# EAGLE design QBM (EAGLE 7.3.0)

## Sheet 1 of 3: dual 1 -> 2 mult
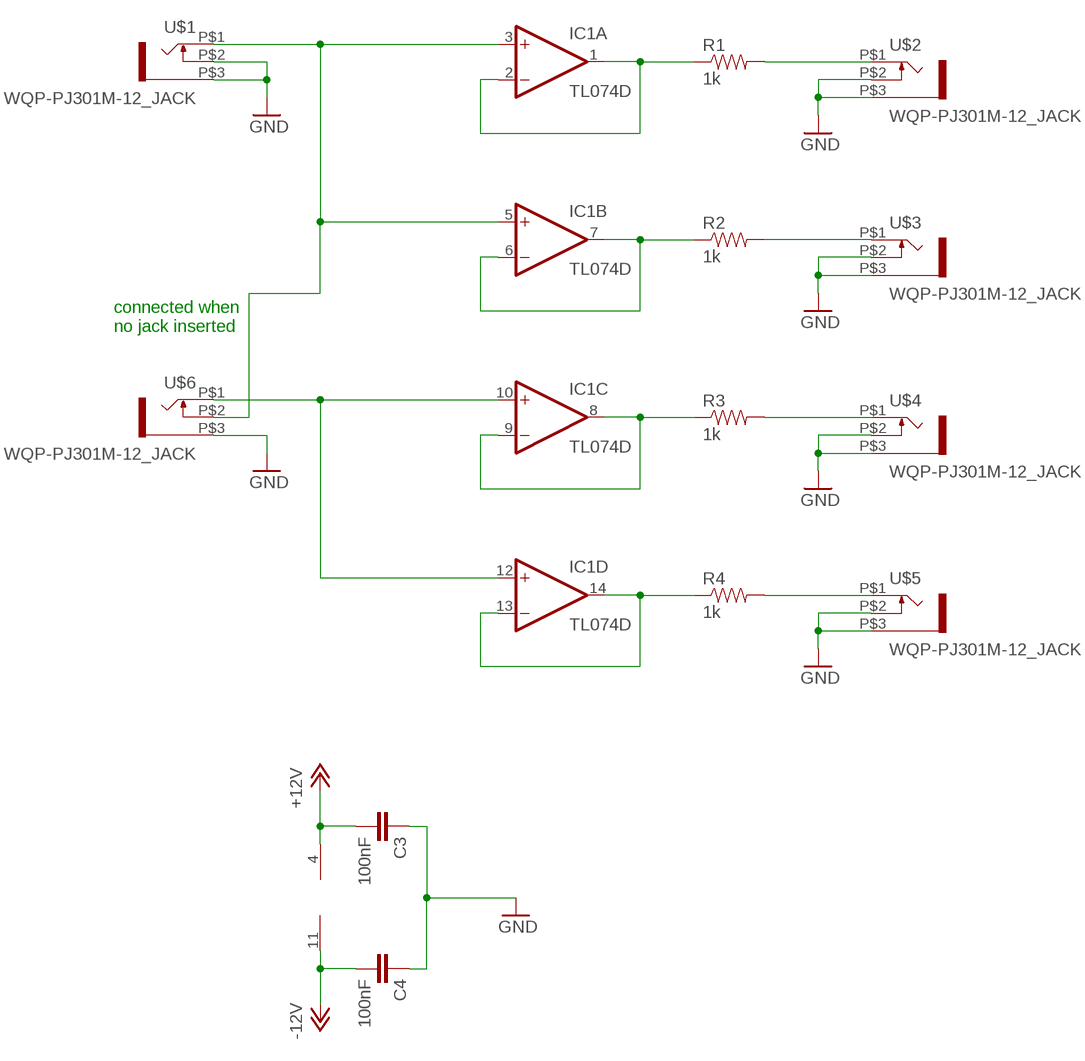
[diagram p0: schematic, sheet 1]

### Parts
C3  100nF  CAP1206  [1206]
C4  100nF  CAP1206  [1206]
IC1  TL074D  [SO14]
R1  1k  RESISTOR1206  [1206]
R2  1k  RESISTOR1206  [1206]
R3  1k  RESISTOR1206  [1206]
R4  1k  RESISTOR1206  [1206]
U$1  WQP-PJ301M-12_JACK  [WQP-PJ301M-12_JACK]
U$2  WQP-PJ301M-12_JACK  [WQP-PJ301M-12_JACK]
U$3  WQP-PJ301M-12_JACK  [WQP-PJ301M-12_JACK]
U$4  WQP-PJ301M-12_JACK  [WQP-PJ301M-12_JACK]
U$5  WQP-PJ301M-12_JACK  [WQP-PJ301M-12_JACK]
U$6  WQP-PJ301M-12_JACK  [WQP-PJ301M-12_JACK]

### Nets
+12V: C3.2 IC1.4(P:V+) ; also sheet 2,3
-12V: C4.2 IC1.11(P:V-) ; also sheet 2,3
GND: C3.1 C4.1 U$1.P$2 U$1.P$3 U$2.P$2 U$2.P$3 U$3.P$2 U$3.P$3 U$4.P$2 U$4.P$3 U$5.P$2 U$5.P$3 U$6.P$3 ; also sheet 2,3
N$3: IC1.3(A:+IN) IC1.5(B:+IN) U$1.P$1 U$6.P$2
N$4: IC1.1(A:OUT) IC1.2(A:-IN) R1.1
N$5: IC1.6(B:-IN) IC1.7(B:OUT) R2.1
N$6: IC1.8(C:OUT) IC1.9(C:-IN) R3.1
N$7: IC1.13(D:-IN) IC1.14(D:OUT) R4.1
N$8: R1.2 U$2.P$1
N$9: R2.2 U$3.P$1
N$10: R3.2 U$4.P$1
N$11: R4.2 U$5.P$1
N$12: IC1.10(C:+IN) IC1.12(D:+IN) U$6.P$1

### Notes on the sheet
- connected when 
  no jack inserted

## Sheet 2 of 3: dual 1 -> 2 mult
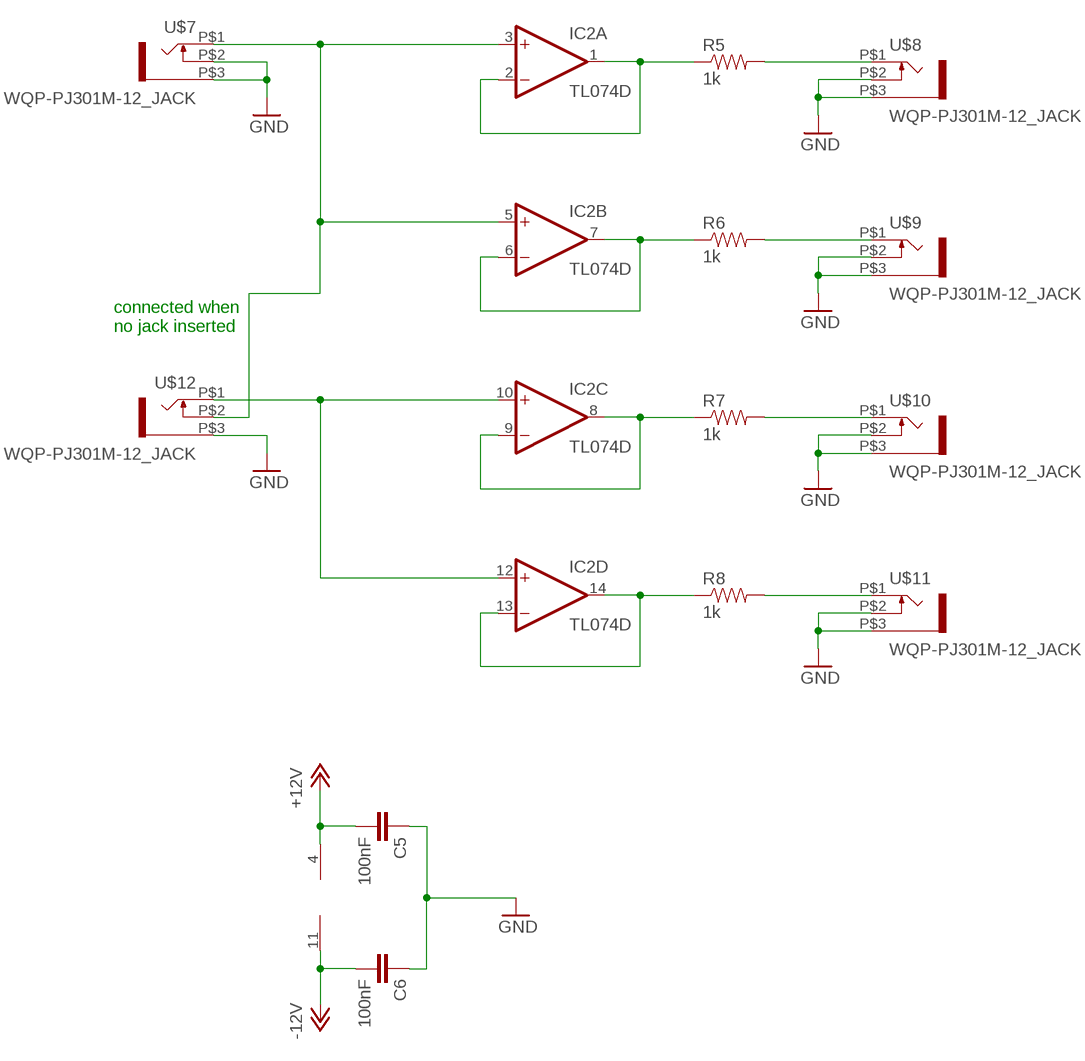
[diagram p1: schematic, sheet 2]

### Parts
C5  100nF  CAP1206  [1206]
C6  100nF  CAP1206  [1206]
IC2  TL074D  [SO14]
R5  1k  RESISTOR1206  [1206]
R6  1k  RESISTOR1206  [1206]
R7  1k  RESISTOR1206  [1206]
R8  1k  RESISTOR1206  [1206]
U$7  WQP-PJ301M-12_JACK  [WQP-PJ301M-12_JACK]
U$8  WQP-PJ301M-12_JACK  [WQP-PJ301M-12_JACK]
U$9  WQP-PJ301M-12_JACK  [WQP-PJ301M-12_JACK]
U$10  WQP-PJ301M-12_JACK  [WQP-PJ301M-12_JACK]
U$11  WQP-PJ301M-12_JACK  [WQP-PJ301M-12_JACK]
U$12  WQP-PJ301M-12_JACK  [WQP-PJ301M-12_JACK]

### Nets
+12V: C5.2 IC2.4(P:V+) ; also sheet 1,3
-12V: C6.2 IC2.11(P:V-) ; also sheet 1,3
GND: C5.1 C6.1 U$7.P$2 U$7.P$3 U$8.P$2 U$8.P$3 U$9.P$2 U$9.P$3 U$10.P$2 U$10.P$3 U$11.P$2 U$11.P$3 U$12.P$3 ; also sheet 1,3
N$13: IC2.3(A:+IN) IC2.5(B:+IN) U$7.P$1 U$12.P$2
N$14: IC2.1(A:OUT) IC2.2(A:-IN) R5.1
N$15: IC2.6(B:-IN) IC2.7(B:OUT) R6.1
N$16: IC2.8(C:OUT) IC2.9(C:-IN) R7.1
N$17: IC2.13(D:-IN) IC2.14(D:OUT) R8.1
N$18: R5.2 U$8.P$1
N$19: R6.2 U$9.P$1
N$20: R7.2 U$10.P$1
N$21: R8.2 U$11.P$1
N$22: IC2.10(C:+IN) IC2.12(D:+IN) U$12.P$1

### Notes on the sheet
- connected when 
  no jack inserted

## Sheet 3 of 3: power
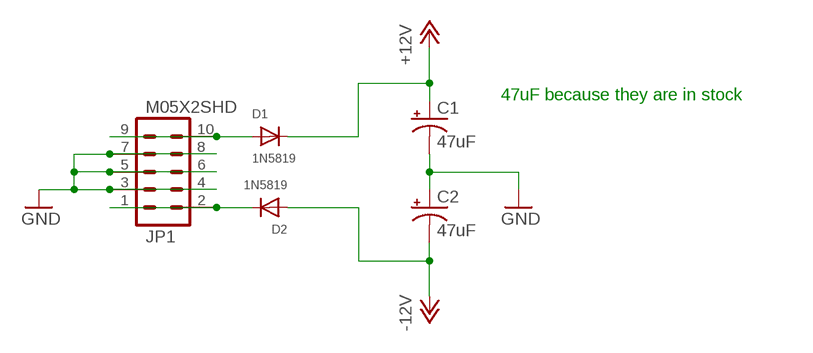
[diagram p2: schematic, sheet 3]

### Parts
C1  47uF  47UF-50V-20%(ELECT)  [PANASONIC_D]
C2  47uF  47UF-50V-20%(ELECT)  [PANASONIC_D]
D1  1N5819  DIODESOD-123  [SOD-123]
D2  1N5819  DIODESOD-123  [SOD-123]
JP1  M05X2SHD  [2X5-SHROUDED]

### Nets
+12V: C1.+ D1.C ; also sheet 1,2
-12V: C2.- D2.A ; also sheet 1,2
GND: C1.- C2.+ JP1.3 JP1.4 JP1.5 JP1.6 JP1.7 JP1.8 ; also sheet 1,2
N$1: D1.A JP1.9 JP1.10
N$2: D2.C JP1.1 JP1.2

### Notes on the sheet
- 47uF because they are in stock

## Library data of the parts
C1 C2 = SparkFun-Capacitors:47UF-50V-20%(ELECT): CAP-10547; PROD_ID: CAP-10547
C3-C6 = SparkFun-Capacitors:CAP: Capacitor
D1 D2 = adafruit:DIODE: Diode
IC1 IC2 = linear:TL074: OP AMP
JP1 = SparkFun:M05X2: Header 5x2 Standard 10-pin dual row 0.1" header. Commonly used with AVR-ISP. Use with Spark Fun Electronics SKU: PRT-00778
R1-R8 = SparkFun:RESISTOR: Resistor
U$1-U$12 = thonkiconn:WQP-PJ301M-12_JACK

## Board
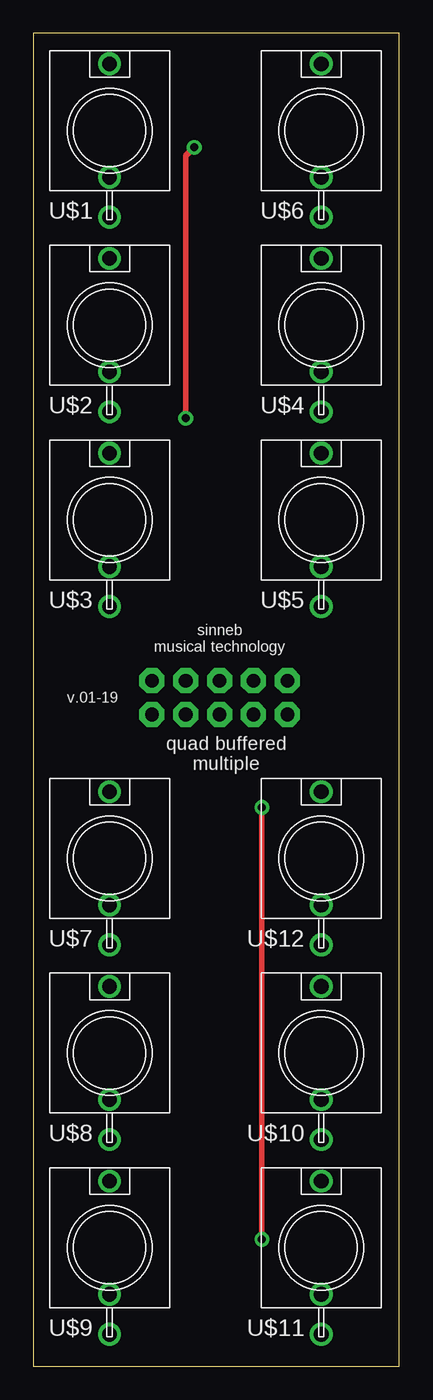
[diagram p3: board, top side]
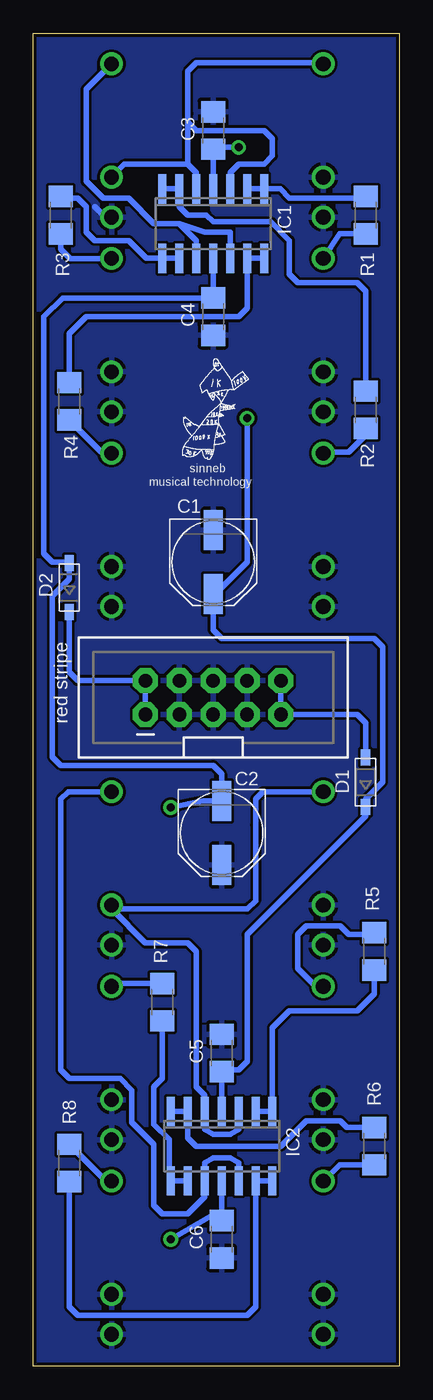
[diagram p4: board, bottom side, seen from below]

Size 27.46 x 100 mm. Coordinates in mm from the lower left corner, seen from the top.
Outline: 0,0 27.46,0 27.46,100 0,100 0,0
Copper layers (1*16): Top 0.035mm / dielectric 1.5mm / Bottom 0.035mm
Design rules "SparkFun": minimum track width 8mil, minimum drill 20mil, track to track 8mil, track to pad 8mil, pad to pad 8mil, via to via 8mil, smd to smd 8mil, copper to edge 10mil, drill to drill 8mil, minimum pad ring 12mil, minimum via ring 10mil, stop-mask expansion 4mil, vias tented up to drill 25mil, thermal gap 10mil

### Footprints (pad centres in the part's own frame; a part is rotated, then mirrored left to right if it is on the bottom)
PANASONIC_D = smd 3 x 1.4: + 2.4,0; - -2.4,0
1206 = smd 1.6 x 1.8: 1 -1.4,0; 2 1.4,0
SOD-123 = smd 1.2 x 0.7: A 1.85,0; C -1.85,0
SO14 = smd 0.6 x 2.2: 1 -3.81,-2.6; 2 -2.54,-2.6; 3 -1.27,-2.6; 4 0,-2.6; 5 1.27,-2.6; 6 2.54,-2.6; 7 3.81,-2.6; 8 3.81,2.6; 9 2.54,2.6; 10 1.27,2.6; 11 0,2.6; 12 -1.27,2.6; 13 -2.54,2.6; 14 -3.81,2.6
2X5-SHROUDED = drill 1.016 pad 1.88 octagon: 1 -1.27,5.08; 2 1.27,5.08; 3 -1.27,2.54; 4 1.27,2.54; 5 -1.27,0; 6 1.27,0; 7 -1.27,-2.54; 8 1.27,-2.54; 9 -1.27,-5.08; 10 1.27,-5.08
WQP-PJ301M-12_JACK = drill 1.1: P$1 0,5; P$2 0,-3.5; P$3 0,-6.5

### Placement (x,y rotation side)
C1  13.97,60.33 270 bottom
C2  13.34,40.01 270 bottom
C3  13.97,92.71 270 bottom
C4  13.97,78.74 90 bottom
C5  13.34,23.5 270 bottom
C6  13.34,9.53 90 bottom
D1  2.54,43.81 90 bottom
D2  24.77,58.42 90 bottom
IC1  13.97,85.72 180 bottom
IC2  13.34,16.51 180 bottom
JP1  13.97,50.16 90 bottom
R1  2.54,86.36 270 bottom
R2  2.54,71.75 270 bottom
R3  25.4,86.36 270 bottom
R4  24.77,72.39 270 bottom
R5  1.9,31.11 90 bottom
R6  1.9,16.51 270 bottom
R7  17.78,27.3 90 bottom
R8  24.77,15.24 90 bottom
U$1  5.71,92.71 0 top
U$2  5.71,78.11 0 top
U$3  5.71,63.5 0 top
U$4  21.59,78.11 0 top
U$5  21.59,63.5 0 top
U$6  21.59,92.71 0 top
U$7  5.71,38.1 0 top
U$8  5.71,23.5 0 top
U$9  5.71,8.89 0 top
U$10  21.59,23.5 0 top
U$11  21.59,8.89 0 top
U$12  21.59,38.1 0 top

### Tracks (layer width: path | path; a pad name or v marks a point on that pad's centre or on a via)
+12V  (via drill 0.6)
  Top 0.406: v11.43,71.12 11.43,90.81 v12.07,91.44
  Bottom 0.406: IC1.4 C3.2 13.84,91.44 v12.07,91.44 | IC2.4 C5.2 13.21,22.23 12.07,22.23 11.43,22.86 11.43,32.38 2.54,41.27 D1.C 2.54,42.55 1.27,43.81 1.27,53.98 1.9,54.61 13.34,54.61 13.97,55.24 C1.+ 13.83,57.92 11.43,60.33 v11.43,71.12
-12V  (via drill 0.6)
  Top 0.406: v17.14,41.91 v17.14,9.53
  Bottom 0.406: IC1.11 C4.2 25.27,80.14 26.67,78.74 26.67,60.96 26.04,60.33 24.82,60.33 D2.A 24.77,59.05 26.04,57.78 26.04,45.72 25.4,45.09 13.97,45.09 13.34,44.45 C2.- 14.75,42.41 v17.14,41.91 | IC2.11 C6.2 13.84,11.43 v17.14,9.53
GND
  Bottom 0.406: U$6.P$3 22.07,86.21 22.86,87
  pour Bottom: 0,0 0,99.69 27.3,99.69 27.3,0
N$1
  Bottom 0.406: JP1.10 JP1.9 3.18,48.9 2.54,48.26 D1.A
N$2
  Bottom 0.406: JP1.1 JP1.2 24.13,51.44 24.77,52.07 D2.C
N$3
  Bottom 0.406: IC1.5 15.24,89.53 | 15.24,89.53 15.88,90.17 | 15.88,90.17 20.63,90.17 U$6.P$2 | 15.88,93.98 15.88,93.34 15.24,92.71 12.7,92.71 10.16,92.71 9.53,92.08 9.53,90.81 10.16,90.17 12.07,90.17 12.7,89.53 IC1.3 | 15.88,93.98 15.88,97.16 15.24,97.79 6.43,97.79 U$1.P$1 | 15.24,89.53 15.88,90.17 | 15.88,90.17 15.88,93.98
N$4
  Bottom 0.406: IC1.2 IC1.1 8.95,88.33 8.26,87.63 2.67,87.63 R1.1
N$5
  Bottom 0.406: IC1.7 IC1.6 16.51,87 15.88,86.36 14.48,86.36 13.97,85.85 9.65,85.85 8.26,84.45 8.26,81.92 7.62,81.28 3.18,81.28 2.54,80.64 R2.1
N$6
  Bottom 0.406: IC1.9 IC1.8 18.99,83.12 20.32,84.45 22.86,84.45 23.5,85.09 23.5,87 24.13,87.63 25.27,87.63 R3.1
N$7
  Bottom 0.406: IC1.14 IC1.13 11.43,79.38 12.07,78.74 23.5,78.74 24.77,77.47 R4.1
N$8
  Bottom 0.406: R1.2 4.49,84.96 U$2.P$1
N$9
  Bottom 0.406: R2.2 2.54,69.85 3.81,68.58 6.27,68.58 U$3.P$1
N$10
  Bottom 0.406: U$4.P$1 24.68,83.11 25.4,83.82 R3.2
N$11
  Bottom 0.406: U$5.P$1 21.67,68.58 22.36,68.58 R4.2
N$12
  Bottom 0.406: IC1.10 15.24,84.45 16.51,85.72 | 16.51,85.72 18.41,85.72 20.32,87.63 22.23,87.63 23.5,88.9 23.5,95.81 U$6.P$1 | IC1.12 12.7,85.09 14.61,85.09 16.51,85.72
N$13
  Bottom 0.406: IC2.3 12.07,17.78 12.7,17.4 13.97,17.4 14.61,17.78 IC2.5 14.61,19.68 14.61,20.32 15.24,20.95 15.24,31.11 15.88,31.75 19.05,31.75 21.59,34.29 U$12.P$2 21.28,34.29 11.43,34.29 10.79,34.92 10.79,40.64 10.79,42.55 10.24,43.1 U$7.P$1
N$14
  Bottom 0.406: R5.1 1.9,27.94 2.54,27.3 3.18,26.67 8.26,26.67 9.53,25.4 IC2.1 IC2.2
N$15
  Bottom 0.406: IC2.7 IC2.6 15.88,17.14 15.24,16.51 8.89,16.51 6.99,18.41 4.45,18.41 3.94,17.91 R6.1
N$16
  Bottom 0.406: IC2.9 IC2.8 17.27,14.04 17.27,17.02 18.41,18.16 18.41,20.95 17.78,21.59 R7.1
N$17
  Bottom 0.406: IC2.14 IC2.13 10.79,4.45 11.43,3.81 24.13,3.81 24.77,4.45 R8.1
N$18
  Bottom 0.406: U$8.P$1 6.27,28.5 7.62,29.84 7.62,32.38 6.99,33.02 4.45,33.02 3.81,32.38 2.04,32.38 R5.2
N$19
  Bottom 0.406: R6.2 4.49,15.11 U$9.P$1
N$20
  Bottom 0.406: R7.2 21.38,28.7 U$10.P$1
N$21
  Bottom 0.406: U$11.P$1 22.02,13.89 R8.2
N$22
  Bottom 0.406: IC2.12 12.07,15.24 12.7,15.62 13.97,15.62 14.61,15.24 | 14.61,15.24 IC2.10 | 14.61,15.24 14.61,12.7 15.88,11.43 17.78,11.43 18.41,12.06 18.41,15.24 18.41,16.51 18.41,16.64 20.07,18.29 20.07,20.7 20.96,21.59 24.77,21.59 25.4,22.23 25.4,42.55 24.84,43.1 U$12.P$1

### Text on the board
tPlace: v.01-19
tNames: sinneb / musical technology | quad buffered / multiple
bNames: sinneb | musical technology | red stripe

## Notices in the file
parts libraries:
SparkFun: Licensing: CC v3.0 Share-Alike You are welcome to use this library for commercial purposes.
SparkFun-Capacitors: Licensing: Creative Commons ShareAlike 4.0 International - https://creativecommons.org/licenses/by-sa/4.0
